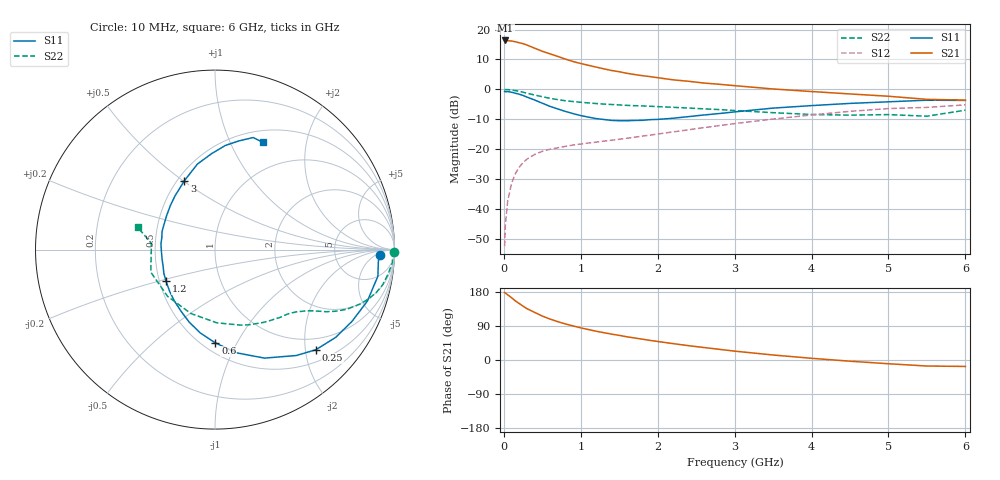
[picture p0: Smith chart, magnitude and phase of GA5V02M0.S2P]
! Infineon Technologies  Discrete & RF Semiconductors
! BF775
! Si NPN RF Bipolar Junction Transistor in SOT23
! VCE = 5 V  IC = 2 mA
! Common Emitter S-Parameters:  May  1996
# GHz  S  MA  R  50
!  f  S11  S21  S12  S22
! GHz  MAG  ANG  MAG  ANG  MAG  ANG  MAG  ANG
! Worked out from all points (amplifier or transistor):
!   36 points, 10 MHz to 6 GHz, reference 50 ohm
!   highest |S21| = 16.3 dB at 20 MHz (marker M1)
!   |S21| within 3 dB of that: start of sweep to 440.6 MHz
!   unconditionally stable (mu >= 1): 1.191 GHz to 3.49 GHz
!   at 250 MHz: K = 0.28, MSG = 19.9 dB, |S12| = -24.5 dB
!   at 1.4 GHz: K = 1.09, MAG = 9.8 dB, |S12| = -17.0 dB
!   at 6 GHz: K = 0.97, MSG = 0.8 dB, |S12| = -5.2 dB
!   S11 on the Smith chart (normalised r, x): 10 MHz: 21, -8; 250 MHz: 0.74, -2.22; 600 MHz: 0.58, -0.82; 1.2 GHz: 0.54, -0.21; 3 GHz: 0.54, +0.51; 6 GHz: 0.64, +1.33
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0.01  0.9209 -1.9  6.557 178.5  0.0024 86.7  0.9977 -0.7
0.02  0.9124 -3.8  6.569 176.6  0.0055 87.4  0.9894 -1.6
0.05  0.9196 -9.3  6.505 172.0  0.0136 84.6  0.9916 -4.1
0.1  0.896 -18.7  6.43 164.4  0.027 79.0  0.9744 -8.0
0.15  0.8615 -27.7  6.249 155.9  0.039 74.1  0.9544 -11.9
0.25  0.7919 -44.8  5.805 142.0  0.0599 65.1  0.8961 -18.0
0.3  0.7439 -52.5  5.508 135.6  0.0682 61.9  0.8632 -20.6
0.4  0.6644 -65.5  4.881 125.7  0.0819 56.2  0.8055 -24.4
0.5  0.5879 -78.1  4.333 115.9  0.0923 52.1  0.7538 -27.1
0.6  0.5199 -89.8  3.928 108.0  0.0999 49.4  0.7094 -29.2
0.7  0.4716 -100.0  3.558 101.2  0.1055 47.8  0.6743 -30.6
0.8  0.4284 -109.7  3.207 95.1  0.1116 46.4  0.6456 -31.9
1  0.3648 -128.4  2.704 84.8  0.1223 45.2  0.6088 -34.1
1.1  0.3437 -137.3  2.523 80.3  0.127 45.4  0.5939 -35.4
1.2  0.325 -147.0  2.357 76.0  0.1314 45.6  0.5801 -36.5
1.6  0.2991 -179.2  1.857 61.2  0.1525 47.5  0.5407 -41.6
2.2  0.3295 144.9  1.444 43.2  0.1947 49.3  0.5018 -51.8
3  0.4203 113.9  1.154 23.4  0.2681 47.1  0.4435 -71.5
3.5  0.4866 101.6  1.016 13.2  0.319 43.1  0.408 -88.6
4.5  0.5832 84.3  0.839 -3.2  0.4296 31.4  0.3709 -135.5
5.5  0.6595 71.2  0.681 -15.9  0.5 15.1  0.3563 174.3
6  0.6544 66.0  0.662 -17.0  0.5512 10.6  0.4493 163.8
